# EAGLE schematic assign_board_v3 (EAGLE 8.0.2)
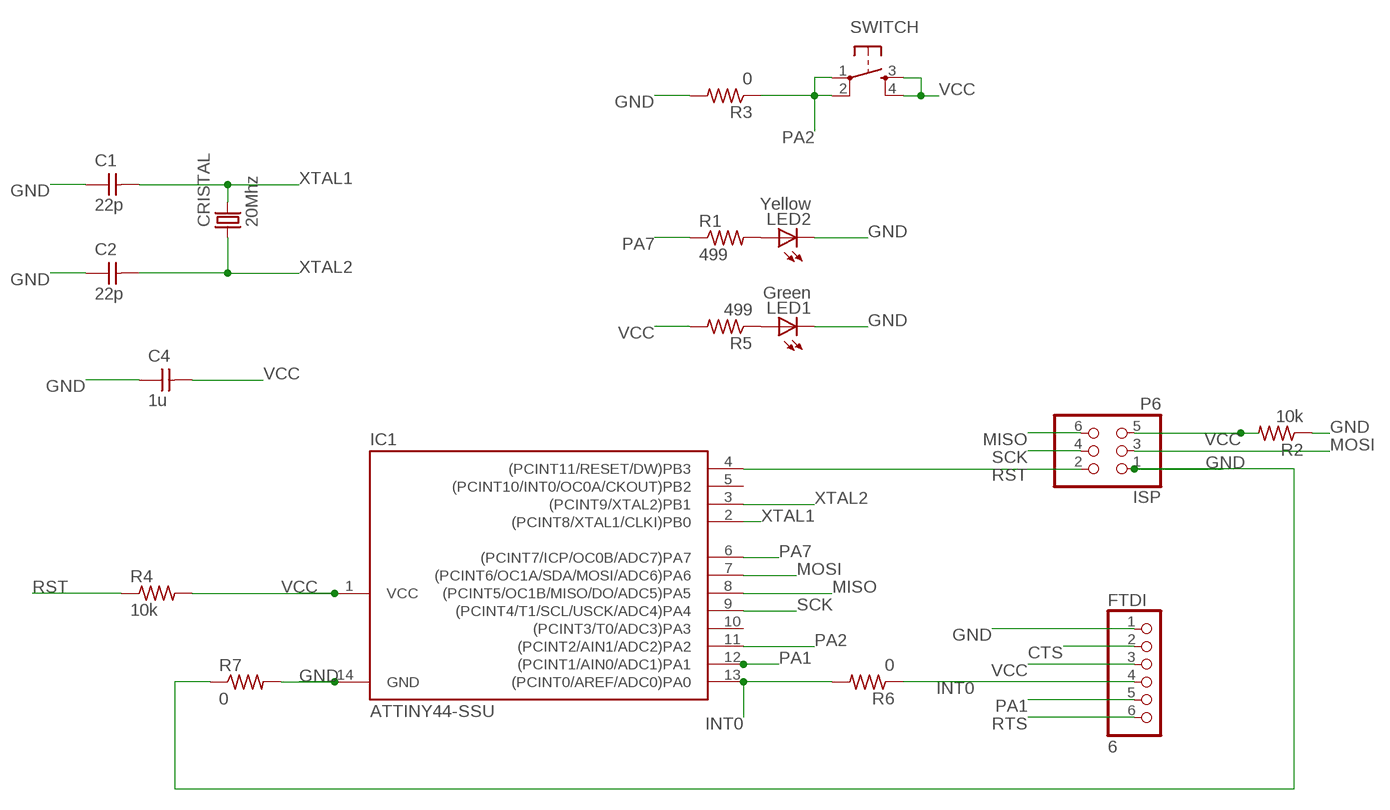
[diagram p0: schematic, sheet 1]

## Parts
C1  22p  CAP-UNPOLARIZED  [C1206]
C2  22p  CAP-UNPOLARIZED  [C1206]
C4  1u  CAP-UNPOLARIZED  [C1206]
CRISTAL  20Mhz  CRYSTAL  [2-SMD-5X3MM]
FTDI  6  PINHD-1X6/90  [1X06/90]
IC1  ATTINY44-SSU  [SOIC14]
ISP  P6  PINHD-2X3-SMD  [2X03SMD]
LED1  Green  LED  [LED1206]
LED2  Yellow  LED  [LED1206]
R1  499  RES-US1206  [R1206]
R2  10k  RES-US1206  [R1206]
R3  0  RES-US1206  [R1206]
R4  10k  RES-US1206  [R1206]
R5  499  RES-US1206  [R1206]
R6  0  RES-US1206  [R1206]
R7  0  RES-US1206  [R1206]
SWITCH  6MM_SWITCH6MM_SWITCH  [6MM_SWITCH]

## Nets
CTS: FTDI.2
GND: C1.1 C2.1 C4.1 FTDI.1 IC1.14(GND) ISP.1 LED1.2(C) LED2.2(C) R2.1 R3.2 R7.1 R7.2
INT0: FTDI.4 IC1.13((PCINT0/AREF/ADC0)PA0) R6.1 R6.2
MISO: IC1.8((PCINT5/OC1B/MISO/DO/ADC5)PA5) ISP.6
MOSI: IC1.7((PCINT6/OC1A/SDA/MOSI/ADC6)PA6) ISP.3
N$1: LED2.1(A) R1.2
N$4: LED1.1(A) R5.1
PA1: FTDI.5 IC1.12((PCINT1/AIN0/ADC1)PA1)
PA2: IC1.11((PCINT2/AIN1/ADC2)PA2) R3.1 SWITCH.1(P) SWITCH.2(P1)
PA7: IC1.6((PCINT7/ICP/OC0B/ADC7)PA7) R1.1
RST: IC1.4((PCINT11/RESET/DW)PB3) ISP.2 R4.1
RTS: FTDI.6
SCK: IC1.9((PCINT4/T1/SCL/USCK/ADC4)PA4) ISP.4
VCC: C4.2 FTDI.3 IC1.1(VCC) ISP.5 R2.2 R4.2 R5.2 SWITCH.3(S) SWITCH.4(S1)
XTAL1: C1.2 CRISTAL.P$2 IC1.2((PCINT8/XTAL1/CLKI)PB0)
XTAL2: C2.2 CRISTAL.P$1 IC1.3((PCINT9/XTAL2)PB1)
Unconnected: IC1.5((PCINT10/INT0/OC0A/CKOUT)PB2) IC1.10((PCINT3/T0/ADC3)PA3)

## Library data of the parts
C1 C2 C4 = fab:CAP-UNPOLARIZED
CRISTAL = fab:CRYSTAL
FTDI = pinhead:PINHD-1X6: PIN HEADER
IC1 = fab:ATTINY44
ISP = fab:PINHD-2X3-SMD: PIN HEADER
LED1 LED2 = fab:LED: LED
R1-R7 = fab:RES-US: Resistor (US Symbol)
SWITCH = fab:6MM_SWITCH: OMRON SWITCH

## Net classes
0 default: clearance 0.205 mm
